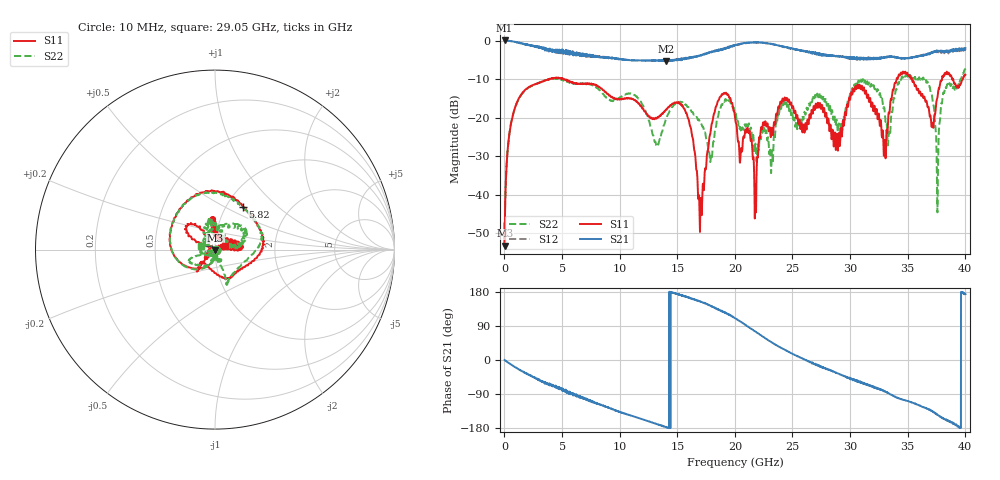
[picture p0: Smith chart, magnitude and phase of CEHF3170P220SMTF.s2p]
!Agilent Technologies,N5224A,MY51441447,A.10.00.00
!Agilent N5224A: A.10.00.00
!Date: Wednesday, January 15, 2020 16:48:35
!Correction: S11(Full 2 Port(1,2))
!S21(Full 2 Port(1,2))
!S12(Full 2 Port(1,2))
!S22(Full 2 Port(1,2))
!S2P File: Measurements: S11, S21, S12, S22:
# Hz S  dB  R 50
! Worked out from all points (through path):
!   4001 points, 10 MHz to 40.01 GHz, reference 50 ohm
!   highest |S21| = 0.01 dB at 10 MHz (marker M1); lowest = -5.3 dB at 14.01 GHz (marker M2)
!   group delay of S21, straight-line fit = 37.1 ps
!   lowest |S11| = -53.3 dB at 20 MHz (marker M3), VSWR 1.00, Z = 50.2 - j0.141 ohm
!   |S11| at or under -10 dB: start of sweep to 3.91 GHz; 5.093 GHz to 34.03 GHz (28.94 GHz wide, 148 % of centre); 35.37 GHz to 37.98 GHz (2.612 GHz wide, 7.12 % of centre)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
!   |S22| runs from -53.4 to -7.4 dB; largest |S21 - S12| = 0.074
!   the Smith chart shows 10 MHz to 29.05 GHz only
!   S11 on the Smith chart (normalised r, x): 10 MHz: 1.01, -0.00; 5.82 GHz: 1.19, +0.62; 29.05 GHz: 1.12, +0.05
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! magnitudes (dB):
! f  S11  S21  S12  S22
! 10 MHz  -47.7  0.0  0.0  -47.1
! 20 MHz  -53.3  0.0  0.0  -53.4
! 1.28 GHz  -14.9  -0.6  -0.6  -14.9
! 5.82 GHz  -10.9  -3.4  -3.1  -11.0
! 6.68 GHz  -11.2  -3.9  -3.8  -11.2
! 13.35 GHz  -20.0  -5.2  -5.3  -27.0
! 14.01 GHz  -17.9  -5.3  -5.2  -20.5
! 15.84 GHz  -19.3  -4.6  -4.7  -17.1
! 16.98 GHz  -47.1  -3.9  -3.9  -21.3
! 18.51 GHz  -15.8  -2.5  -2.5  -20.0
! 20.01 GHz  -19.8  -1.2  -1.3  -19.0
! 21.75 GHz  -40.5  -0.5  -0.5  -27.3
! 24.13 GHz  -15.1  -1.5  -1.6  -16.5
! 26.68 GHz  -18.1  -3.0  -3.2  -16.1
! 29.05 GHz  -24.1  -4.1  -4.1  -21.8
! 31.09 GHz  -13.0  -4.7  -4.9  -10.3
! 33.35 GHz  -18.8  -4.2  -4.1  -24.4
! 34.43 GHz  -8.3  -4.6  -4.5  -10.1
! 36.35 GHz  -14.8  -3.9  -3.6  -9.6
! 37.59 GHz  -14.7  -2.8  -3.0  -43.0
! 38.22 GHz  -8.5  -2.8  -3.0  -12.6
! 40.01 GHz  -8.9  -2.0  -2.5  -7.6
